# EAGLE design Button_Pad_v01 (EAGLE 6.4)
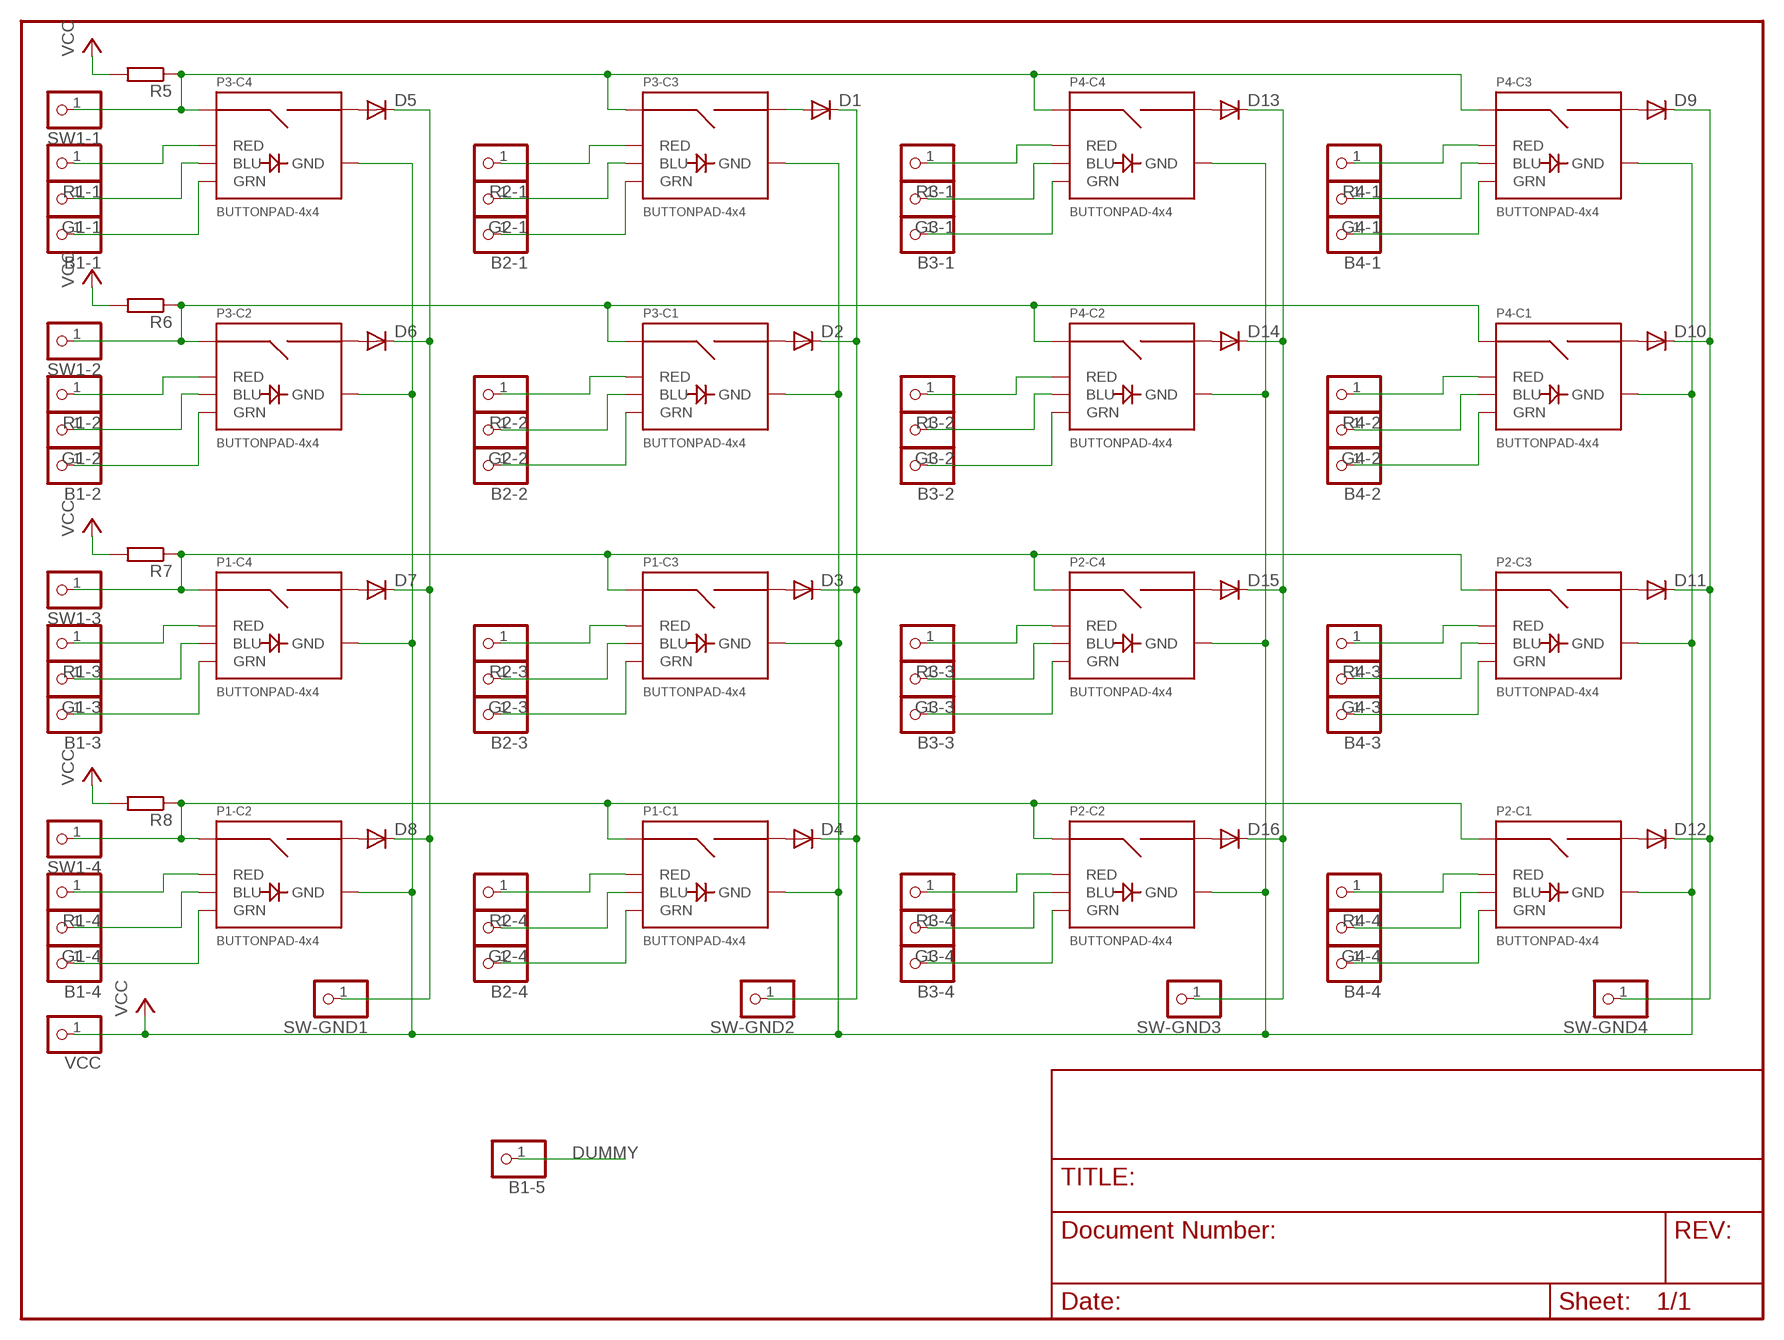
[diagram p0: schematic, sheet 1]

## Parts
B1-1  PINHD-1X1  [1X01]
B1-2  PINHD-1X1  [1X01]
B1-3  PINHD-1X1  [1X01]
B1-4  PINHD-1X1  [1X01]
B1-5  PINHD-1X1  [1X01]
B2-1  PINHD-1X1  [1X01]
B2-2  PINHD-1X1  [1X01]
B2-3  PINHD-1X1  [1X01]
B2-4  PINHD-1X1  [1X01]
B3-1  PINHD-1X1  [1X01]
B3-2  PINHD-1X1  [1X01]
B3-3  PINHD-1X1  [1X01]
B3-4  PINHD-1X1  [1X01]
B4-1  PINHD-1X1  [1X01]
B4-2  PINHD-1X1  [1X01]
B4-3  PINHD-1X1  [1X01]
B4-4  PINHD-1X1  [1X01]
D1  DIODE-1N4148  [DOIDE-1N4148]
D2  DIODE-1N4148  [DOIDE-1N4148]
D3  DIODE-1N4148  [DOIDE-1N4148]
D4  DIODE-1N4148  [DOIDE-1N4148]
D5  DIODE-1N4148  [DOIDE-1N4148]
D6  DIODE-1N4148  [DOIDE-1N4148]
D7  DIODE-1N4148  [DOIDE-1N4148]
D8  DIODE-1N4148  [DOIDE-1N4148]
D9  DIODE-1N4148  [DOIDE-1N4148]
D10  DIODE-1N4148  [DOIDE-1N4148]
D11  DIODE-1N4148  [DOIDE-1N4148]
D12  DIODE-1N4148  [DOIDE-1N4148]
D13  DIODE-1N4148  [DOIDE-1N4148]
D14  DIODE-1N4148  [DOIDE-1N4148]
D15  DIODE-1N4148  [DOIDE-1N4148]
D16  DIODE-1N4148  [DOIDE-1N4148]
G1-1  PINHD-1X1  [1X01]
G1-2  PINHD-1X1  [1X01]
G1-3  PINHD-1X1  [1X01]
G1-4  PINHD-1X1  [1X01]
G2-1  PINHD-1X1  [1X01]
G2-2  PINHD-1X1  [1X01]
G2-3  PINHD-1X1  [1X01]
G2-4  PINHD-1X1  [1X01]
G3-1  PINHD-1X1  [1X01]
G3-2  PINHD-1X1  [1X01]
G3-3  PINHD-1X1  [1X01]
G3-4  PINHD-1X1  [1X01]
G4-1  PINHD-1X1  [1X01]
G4-2  PINHD-1X1  [1X01]
G4-3  PINHD-1X1  [1X01]
G4-4  PINHD-1X1  [1X01]
P1  BUTTONPAD-4x4  BUTTONPAD-2X2  [BUTTONPAD-2X2]
P2  BUTTONPAD-4x4  BUTTONPAD-2X2  [BUTTONPAD-2X2]
P3  BUTTONPAD-4x4  BUTTONPAD-2X2  [BUTTONPAD-2X2]
P4  BUTTONPAD-4x4  BUTTONPAD-2X2  [BUTTONPAD-2X2]
R1-1  PINHD-1X1  [1X01]
R1-2  PINHD-1X1  [1X01]
R1-3  PINHD-1X1  [1X01]
R1-4  PINHD-1X1  [1X01]
R2-1  PINHD-1X1  [1X01]
R2-2  PINHD-1X1  [1X01]
R2-3  PINHD-1X1  [1X01]
R2-4  PINHD-1X1  [1X01]
R3-1  PINHD-1X1  [1X01]
R3-2  PINHD-1X1  [1X01]
R3-3  PINHD-1X1  [1X01]
R3-4  PINHD-1X1  [1X01]
R4-1  PINHD-1X1  [1X01]
R4-2  PINHD-1X1  [1X01]
R4-3  PINHD-1X1  [1X01]
R4-4  PINHD-1X1  [1X01]
R5  R-EU_0204/7  [0204/7]
R6  R-EU_0204/7  [0204/7]
R7  R-EU_0204/7  [0204/7]
R8  R-EU_0204/7  [0204/7]
SW1-1  PINHD-1X1  [1X01]
SW1-2  PINHD-1X1  [1X01]
SW1-3  PINHD-1X1  [1X01]
SW1-4  PINHD-1X1  [1X01]
SW-GND1  PINHD-1X1  [1X01]
SW-GND2  PINHD-1X1  [1X01]
SW-GND3  PINHD-1X1  [1X01]
SW-GND4  PINHD-1X1  [1X01]
VCC  PINHD-1X1  [1X01]

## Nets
DUMMY: B1-5.1
G3-2: G3-2.1 P4.BLU2(-C2:BLU)
N$1: D1.P$1(A) P3.SIG6(-C3:SIG2)
N$2: D2.P$1(A) P3.SIG2(-C1:SIG2)
N$3: D3.P$1(A) P1.SIG6(-C3:SIG2)
N$4: D4.P$1(A) P1.SIG2(-C1:SIG2)
N$5: D5.P$1(A) P3.SIG8(-C4:SIG2)
N$6: D6.P$1(A) P3.SIG4(-C2:SIG2)
N$7: D7.P$1(A) P1.SIG8(-C4:SIG2)
N$8: D8.P$1(A) P1.SIG4(-C2:SIG2)
N$9: D9.P$1(A) P4.SIG6(-C3:SIG2)
N$10: D10.P$1(A) P4.SIG2(-C1:SIG2)
N$11: D11.P$1(A) P2.SIG6(-C3:SIG2)
N$12: D12.P$1(A) P2.SIG2(-C1:SIG2)
N$13: D13.P$1(A) P4.SIG8(-C4:SIG2)
N$14: D14.P$1(A) P4.SIG4(-C2:SIG2)
N$15: D15.P$1(A) P2.SIG8(-C4:SIG2)
N$16: D16.P$1(A) P2.SIG4(-C2:SIG2)
N$17: B4-1.1 P4.GRN3(-C3:GRN)
N$18: G4-1.1 P4.BLU3(-C3:BLU)
N$19: P4.RED3(-C3:RED) R4-1.1
N$20: B4-2.1 P4.GRN1(-C1:GRN)
N$21: G4-2.1 P4.BLU1(-C1:BLU)
N$22: P4.RED1(-C1:RED) R4-2.1
N$23: P2.RED3(-C3:RED) R4-3.1
N$24: G4-3.1 P2.BLU3(-C3:BLU)
N$25: B4-3.1 P2.GRN3(-C3:GRN)
N$26: P3.RED4(-C4:RED) R1-1.1
N$27: B4-4.1 P2.GRN1(-C1:GRN)
N$28: G4-4.1 P2.BLU1(-C1:BLU)
N$29: P2.RED1(-C1:RED) R4-4.1
N$30: G1-1.1 P3.BLU4(-C4:BLU)
N$31: B1-1.1 P3.GRN4(-C4:GRN)
N$32: P2.RED2(-C2:RED) R3-4.1
N$33: B3-4.1 P2.GRN2(-C2:GRN)
N$34: G3-4.1 P2.BLU2(-C2:BLU)
N$35: B2-4.1 P1.GRN1(-C1:GRN)
N$36: G2-4.1 P1.BLU1(-C1:BLU)
N$37: P1.RED1(-C1:RED) R2-4.1
N$38: P1.RED2(-C2:RED) R1-4.1
N$39: G1-4.1 P1.BLU2(-C2:BLU)
N$40: B1-4.1 P1.GRN2(-C2:GRN)
N$41: B1-3.1 P1.GRN4(-C4:GRN)
N$42: G1-3.1 P1.BLU4(-C4:BLU)
N$43: P1.RED4(-C4:RED) R1-3.1
N$44: B1-2.1 P3.GRN2(-C2:GRN)
N$45: G1-2.1 P3.BLU2(-C2:BLU)
N$46: P3.RED2(-C2:RED) R1-2.1
N$47: P3.RED3(-C3:RED) R2-1.1
N$48: G2-1.1 P3.BLU3(-C3:BLU)
N$49: B2-1.1 P3.GRN3(-C3:GRN)
N$50: B2-2.1 P3.GRN1(-C1:GRN)
N$51: G2-2.1 P3.BLU1(-C1:BLU)
N$52: P3.RED1(-C1:RED) R2-2.1
N$53: B2-3.1 P1.GRN3(-C3:GRN)
N$54: G2-3.1 P1.BLU3(-C3:BLU)
N$55: P1.RED3(-C3:RED) R2-3.1
N$56: B3-3.1 P2.GRN4(-C4:GRN)
N$57: G3-3.1 P2.BLU4(-C4:BLU)
N$58: P2.RED4(-C4:RED) R3-3.1
N$59: B3-2.1 P4.GRN2(-C2:GRN)
N$61: P4.RED2(-C2:RED) R3-2.1
N$62: B3-1.1 P4.GRN4(-C4:GRN)
N$63: G3-1.1 P4.BLU4(-C4:BLU)
N$64: P4.RED4(-C4:RED) R3-1.1
SW2-1: P3.SIG5(-C3:SIG1) P3.SIG7(-C4:SIG1) P4.SIG5(-C3:SIG1) P4.SIG7(-C4:SIG1) R5.1 SW1-1.1
SW2-2: P3.SIG1(-C1:SIG1) P3.SIG3(-C2:SIG1) P4.SIG1(-C1:SIG1) P4.SIG3(-C2:SIG1) R6.1 SW1-2.1
SW2-3: P1.SIG5(-C3:SIG1) P1.SIG7(-C4:SIG1) P2.SIG5(-C3:SIG1) P2.SIG7(-C4:SIG1) R7.1 SW1-3.1
SW2-4: P1.SIG1(-C1:SIG1) P1.SIG3(-C2:SIG1) P2.SIG1(-C1:SIG1) P2.SIG3(-C2:SIG1) R8.1 SW1-4.1
SWT-GND1 [ButtonSignal]: D1.P$2(C) D2.P$2(C) D3.P$2(C) D4.P$2(C) SW-GND2.1
SWT-GND2 [ButtonSignal]: D5.P$2(C) D6.P$2(C) D7.P$2(C) D8.P$2(C) SW-GND1.1
SWT-GND3 [ButtonSignal]: D9.P$2(C) D10.P$2(C) D11.P$2(C) D12.P$2(C) SW-GND4.1
SWT-GND4 [ButtonSignal]: D13.P$2(C) D14.P$2(C) D15.P$2(C) D16.P$2(C) SW-GND3.1
VCC: P1.GND1(-C1:GND) P1.GND2(-C2:GND) P1.GND3(-C3:GND) P1.GND4(-C4:GND) P2.GND1(-C1:GND) P2.GND2(-C2:GND) P2.GND3(-C3:GND) P2.GND4(-C4:GND) P3.GND1(-C1:GND) P3.GND2(-C2:GND) P3.GND3(-C3:GND) P3.GND4(-C4:GND) P4.GND1(-C1:GND) P4.GND2(-C2:GND) P4.GND3(-C3:GND) P4.GND4(-C4:GND) R5.2 R6.2 R7.2 R8.2 VCC.1

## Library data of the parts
B1-1-B1-5 B2-1-B2-4 B3-1-B3-4 B4-1-B4-4 G1-1-G1-4 G2-1-G2-4 G3-1-G3-4 G4-1-G4-4 R1-1-R1-4 R2-1-R2-4 R3-1-R3-4 R4-1-R4-4 SW1-1-SW1-4 SW-GND1-SW-GND4 VCC = pinhead:PINHD-1X1: PIN HEADER
D1-D16 = SparkFun:DIODE-1N4148
P1-P4 = SparkFun:BUTTONPAD-2X2: 5mm Button Pad Proven layout and schematic for 2x2 button pad. Panelize this device/fp to a 4x4 pad if needed. Spark Fun Electronics SKU : COM-07835. Compatible common cathode tri-color LED SKU : COM-00105
R5-R8 = rcl:R-EU_: RESISTOR, European symbol

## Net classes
0 Default: width 0.254 mm, clearance 0.355 mm
1 Power: width 0.305 mm
2 LEDPower: width 0.305 mm
3 ButtonSignal: width 0.254 mm, clearance 0.355 mm to class 0, clearance 0.355 mm to class 1, clearance 0.355 mm to class 2, clearance 0.355 mm

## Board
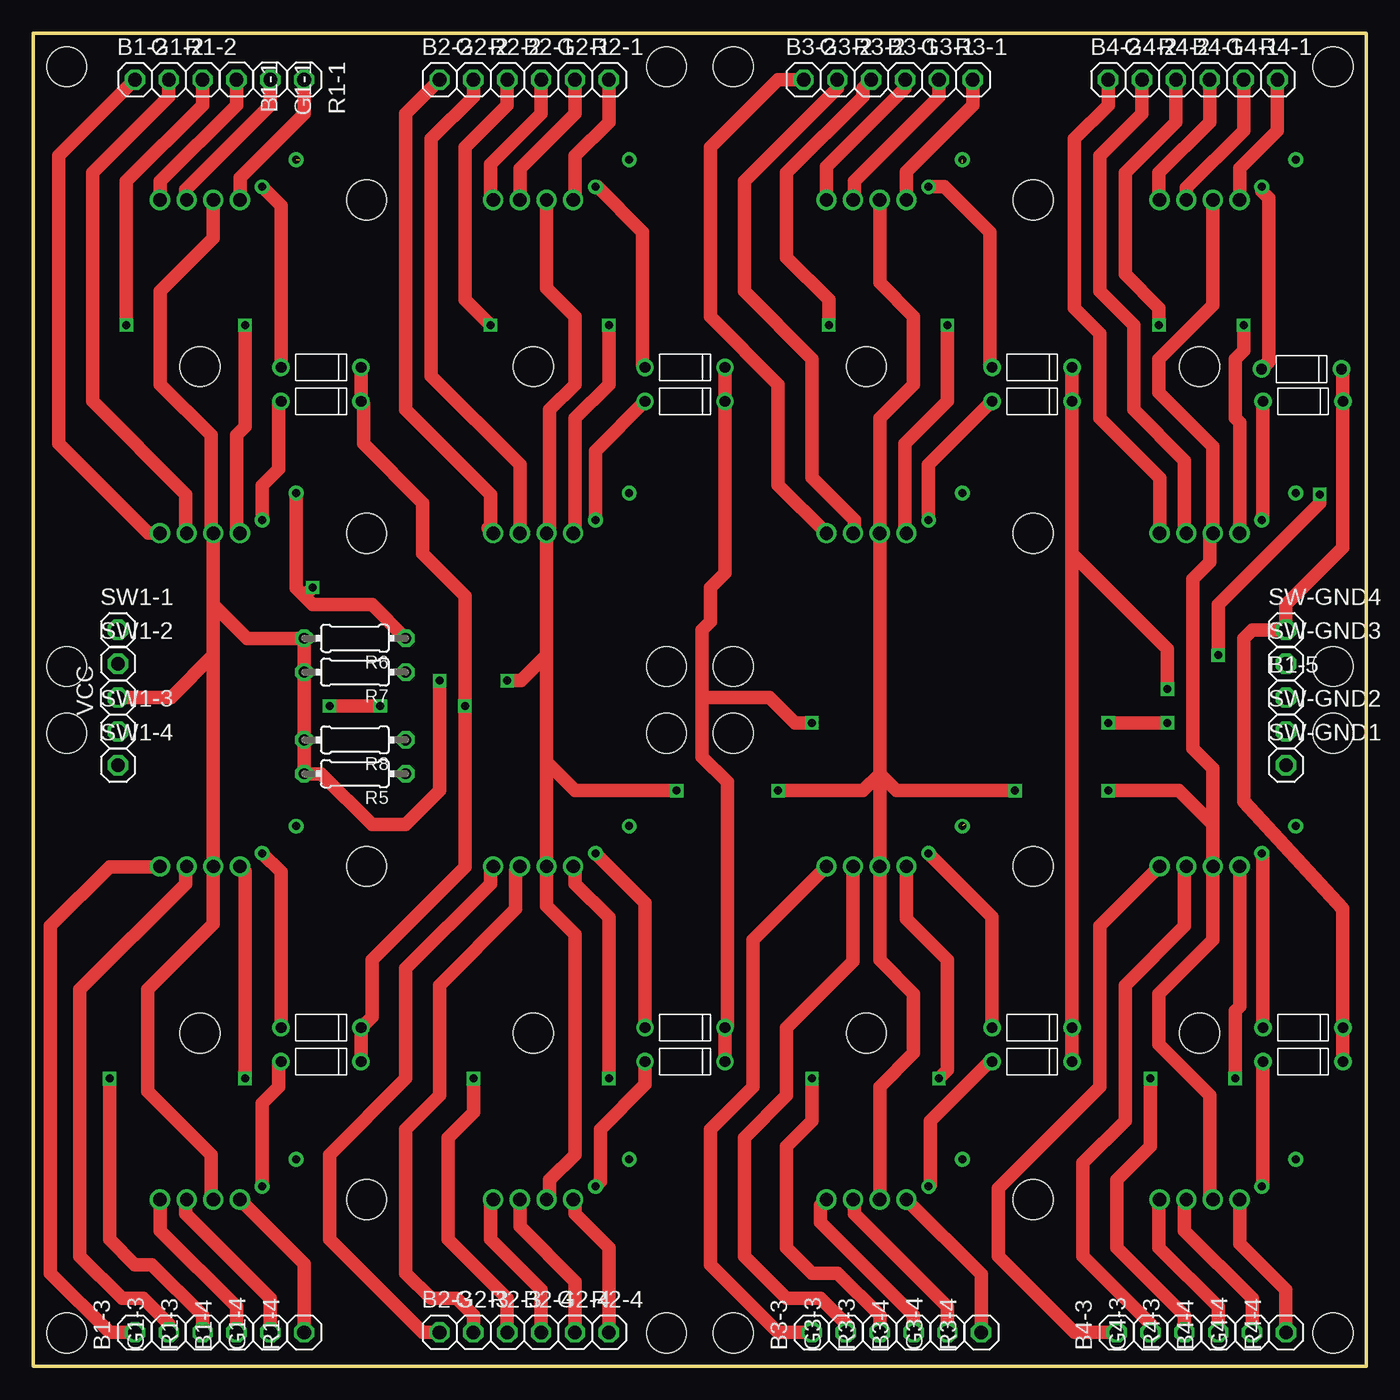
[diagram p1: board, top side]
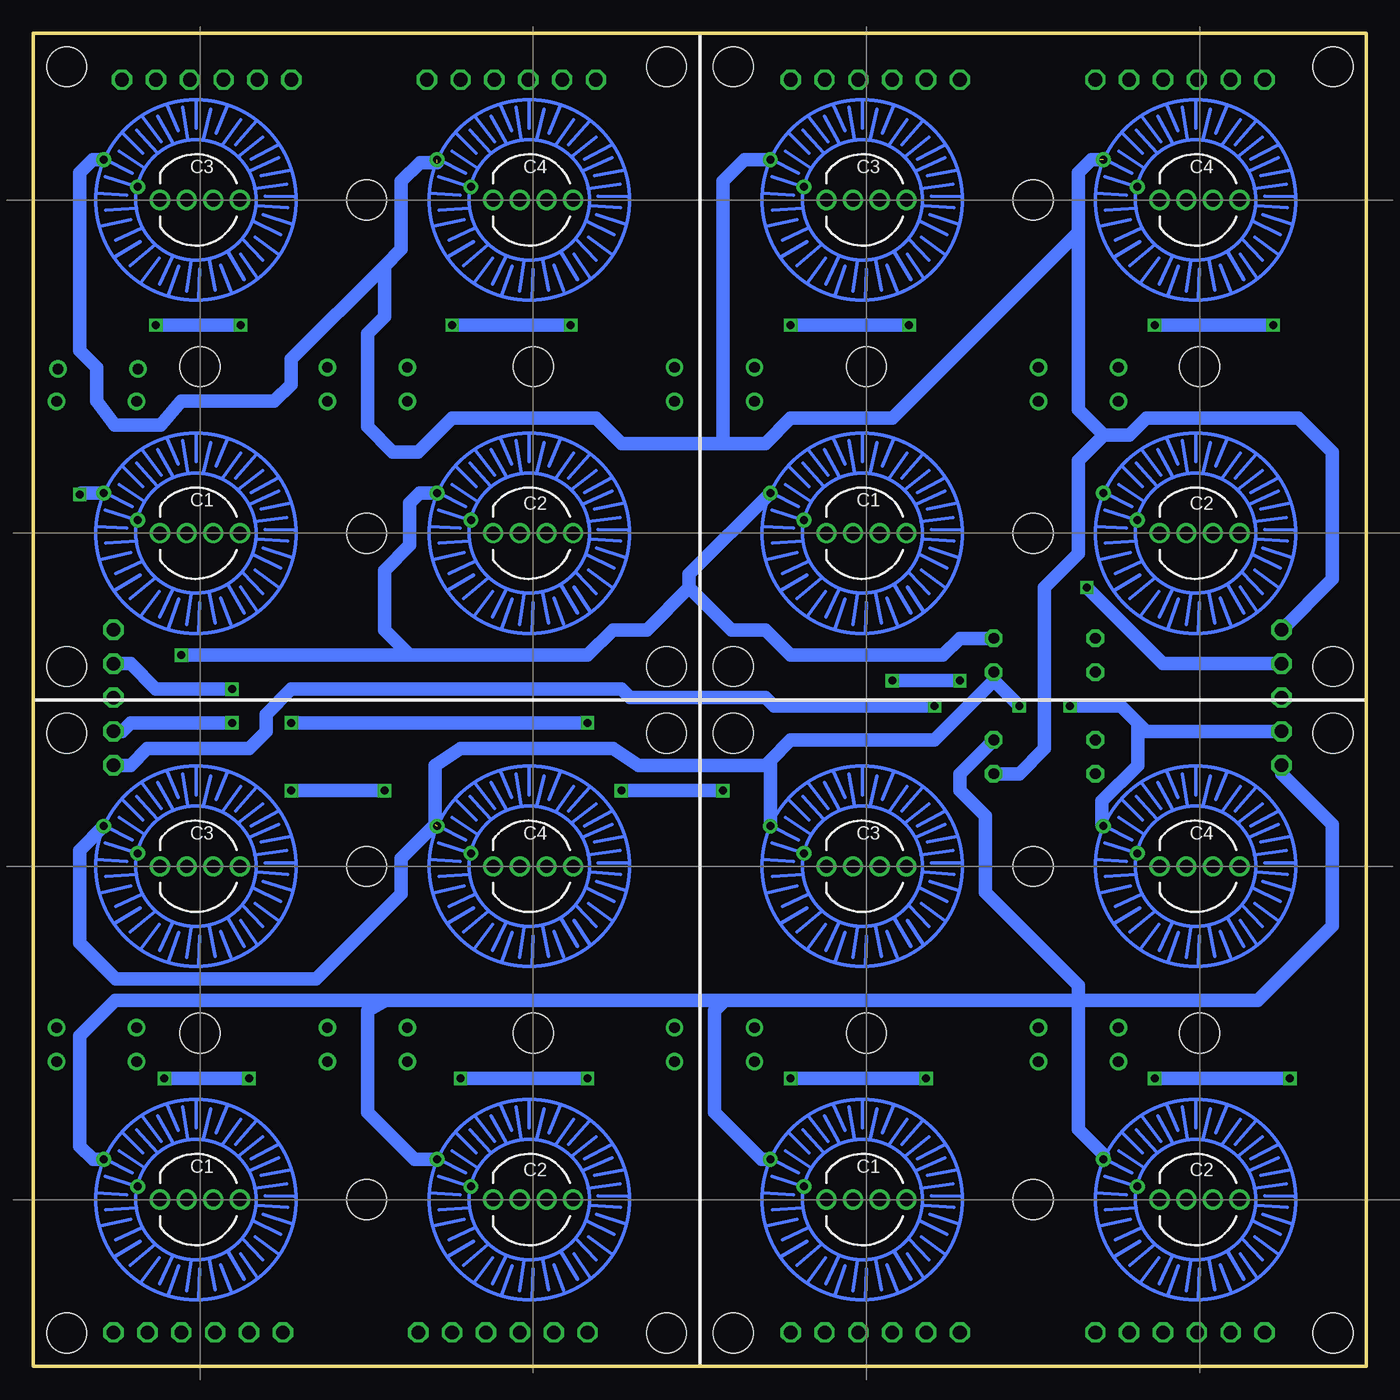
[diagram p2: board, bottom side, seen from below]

Size 100 x 100 mm. Coordinates in mm from the lower left corner, seen from the top.
Outline: 0,0 100,0 100,100 0,100 0,0
Copper layers (1*16): Top 0.035mm / dielectric 1.5mm / Bottom 0.035mm
Design rules "default *": minimum track width 7mil, minimum drill 20mil, track to track 7mil, track to pad 7mil, pad to pad 7mil, via to via 7mil, smd to smd 7mil, copper to edge 20mil, drill to drill 7mil, minimum pad ring 10mil, minimum via ring 8mil, stop-mask expansion 4mil, vias tented up to drill 0mil, thermal gap 10mil

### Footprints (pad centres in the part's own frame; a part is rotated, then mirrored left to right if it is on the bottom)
1X01 = drill 1.016 octagon: 1 0,0
DOIDE-1N4148 = drill 0.8: P$1 3,0; P$2 -3,0
BUTTONPAD-2X2 = drill 1: BLU1 13.5,12.5; BLU2 38.5,12.5; BLU3 13.5,37.5; BLU4 38.5,37.5; GND1 11.5,12.5; GND2 36.5,12.5; GND3 11.5,37.5; GND4 36.5,37.5; GRN1 15.5,12.5; GRN2 40.5,12.5; GRN3 15.5,37.5; GRN4 40.5,37.5; RED1 9.5,12.5; RED2 34.5,12.5; RED3 9.5,37.5; RED4 34.5,37.5 | drill 0.6: SIG1 5.288,15.513; SIG2 7.828,13.481; SIG3 30.288,15.513; SIG4 32.828,13.481; SIG5 5.288,40.513; SIG6 7.828,38.481; SIG7 30.288,40.513; SIG8 32.828,38.481 | hole 3: 12.5,25; 25,37.5; 37.5,25; 25,12.5; 2.5,2.5; 2.5,47.5; 47.5,47.5; 47.5,2.5
0204/7 = drill 0.813 octagon: 1 -3.81,0; 2 3.81,0

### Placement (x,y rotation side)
B1-1  15.24,96.52 270 top
B1-2  7.62,96.52 0 top
B1-3  7.62,2.54 90 top
B1-4  15.24,2.54 90 top
B1-5  93.98,50.16 0 top
B2-1  38.1,96.52 0 top
B2-2  30.48,96.52 0 top
B2-3  30.48,2.54 0 top
B2-4  38.1,2.54 0 top
B3-1  65.41,96.52 0 top
B3-2  57.78,96.52 0 top
B3-3  58.42,2.54 90 top
B3-4  66.04,2.54 90 top
B4-1  88.27,96.52 0 top
B4-2  80.64,96.52 0 top
B4-3  81.28,2.54 90 top
B4-4  88.9,2.54 90 top
D1  48.9,74.93 180 top
D2  48.9,72.39 180 top
D3  48.9,25.4 180 top
D4  48.9,22.86 180 top
D5  21.59,74.93 180 top
D6  21.59,72.39 180 top
D7  21.59,25.4 180 top
D8  21.59,22.86 180 top
D9  95.15,74.81 180 top
D10  95.25,72.39 180 top
D11  95.25,25.4 180 top
D12  95.25,22.86 180 top
D13  74.93,74.93 180 top
D14  74.93,72.39 180 top
D15  74.93,25.4 180 top
D16  74.93,22.86 180 top
G1-1  17.78,96.52 270 top
G1-2  10.16,96.52 0 top
G1-3  10.16,2.54 90 top
G1-4  17.78,2.54 90 top
G2-1  40.64,96.52 0 top
G2-2  33.02,96.52 0 top
G2-3  33.02,2.54 0 top
G2-4  40.64,2.54 0 top
G3-1  67.94,96.52 0 top
G3-2  60.33,96.52 0 top
G3-3  60.96,2.54 90 top
G3-4  68.58,2.54 90 top
G4-1  90.81,96.52 0 top
G4-2  83.19,96.52 0 top
G4-3  83.82,2.54 90 top
G4-4  91.44,2.54 90 top
P1  50,0 0 bottom
P2  100,0 0 bottom
P3  50,50 0 bottom
P4  100,50 0 bottom
R1-1  20.32,96.52 270 top
R1-2  12.7,96.52 0 top
R1-3  12.7,2.54 90 top
R1-4  20.32,2.54 90 top
R2-1  43.18,96.52 0 top
R2-2  35.56,96.52 0 top
R2-3  35.56,2.54 0 top
R2-4  43.18,2.54 0 top
R3-1  70.48,96.52 0 top
R3-2  62.87,96.52 0 top
R3-3  63.5,2.54 90 top
R3-4  71.12,2.54 90 top
R4-1  93.34,96.52 0 top
R4-2  85.72,96.52 0 top
R4-3  86.36,2.54 90 top
R4-4  93.98,2.54 90 top
R5  24.13,44.45 180 top
R6  24.13,54.61 180 top
R7  24.13,52.07 180 top
R8  24.13,46.99 180 top
SW1-1  6.35,55.24 0 top
SW1-2  6.35,52.7 0 top
SW1-3  6.35,47.62 0 top
SW1-4  6.35,45.09 0 top
SW-GND1  93.98,45.09 0 top
SW-GND2  93.98,47.62 0 top
SW-GND3  93.98,52.7 0 top
SW-GND4  93.98,55.24 0 top
VCC  6.35,50.16 90 top

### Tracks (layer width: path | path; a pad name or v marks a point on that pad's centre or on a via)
G3-2
  Top 1.016: P4.BLU2 61.59,62.59 61.59,63.5 58.42,66.67 58.42,75.56 53.34,80.64 53.34,88.9 60.33,95.89 G3-2.1
N$1
  Top 1.016: P3.SIG6 42.33,88.48 45.72,85.09 45.72,75.11 D1.P$1
N$2
  Top 1.016: P3.SIG2 42.17,68.67 D2.P$1
N$3
  Top 1.016: D3.P$1 45.9,34.76 P1.SIG6
N$4
  Top 1.016: D4.P$1 45.9,21.13 42.55,17.78 42.55,13.85 P1.SIG2
N$5
  Top 1.016: D5.P$1 18.59,87.06 P3.SIG8
N$6
  Top 1.016: P3.SIG4 17.17,66.07 18.41,67.31 18.41,72.22 D6.P$1
N$7
  Top 1.016: D7.P$1 18.59,37.06 P1.SIG8
N$8
  Top 1.016: P1.SIG4 17.17,19.71 18.41,20.95 18.41,22.68 D8.P$1
N$9
  Top 1.016: P4.SIG6 92.17,88.17 92.71,87.63 92.71,75.37 D9.P$1
N$10
  Top 1.016: D10.P$1 92.25,63.56 P4.SIG2
N$11
  Top 1.016: D11.P$1 92.25,38.4 P2.SIG6
N$12
  Top 1.016: D12.P$1 92.25,13.56 P2.SIG2
N$13
  Top 1.016: P4.SIG8 68.36,88.48 71.75,85.09 71.75,75.11 D13.P$1
N$14
  Top 1.016: P4.SIG4 67.17,67.63 D14.P$1
N$15
  Top 1.016: D15.P$1 71.93,33.72 P2.SIG8
N$16
  Top 1.016: D16.P$1 71.75,22.86 67.31,18.41 67.31,13.62 P2.SIG4
N$17
  Top 1.016: B4-1.1 88.27,93.34 84.45,89.53 84.45,87.55 P4.GRN3
N$18
  Top 1.016: P4.BLU3 86.5,88.41 90.81,92.71 G4-1.1
N$19
  Top 1.016: P4.RED3 90.5,89.86 93.34,92.71 R4-1.1
N$20
  Top 1.016: P4.GRN1 84.5,66.63 80.01,71.12 80.01,77.47 78.11,79.38 78.11,92.08 80.64,94.61 B4-2.1
N$21
  Top 1.016: P4.BLU1 86.36,62.64 86.36,67.94 82.55,71.75 82.55,78.11 80.01,80.64 80.01,90.81 83.19,93.98 G4-2.1
N$22  (via drill 0.6)
  Top 1.016: R4-2.1 85.72,93.34 81.92,89.53 81.92,81.92 84.45,79.38 v84.45,78.11 | v90.81,78.11 90.81,76.2 90.17,75.56 90.17,71.12 90.5,70.79 P4.RED1
  Bottom 1.016: v84.45,78.11 v90.81,78.11
N$23  (via drill 0.6)
  Top 1.016: R4-3.1 86.36,3.81 81.28,8.89 81.28,13.97 83.82,16.51 v83.82,21.59 | P2.RED3 90.5,27 90.17,26.67 v90.17,21.59
  Bottom 1.016: v83.82,21.59 v90.17,21.59
N$24
  Top 1.016: G4-3.1 83.82,3.17 78.74,8.26 78.74,15.24 81.92,18.41 81.92,28.57 86.36,33.02 86.36,37.36 P2.BLU3
N$25
  Top 1.016: P2.GRN3 80.01,33.02 80.01,20.95 72.39,13.34 72.39,8.26 78.11,2.54 B4-3.1
N$26
  Top 1.016: R1-1.1 20.32,93.98 15.5,89.16 P3.RED4
N$27
  Top 1.016: P2.GRN1 84.45,12.46 84.45,8.89 88.9,4.45 B4-4.1
N$28
  Top 1.016: G4-4.1 91.44,5.08 86.36,10.16 86.36,12.36 P2.BLU1
N$29
  Top 1.016: R4-4.1 93.98,5.71 90.5,9.2 P2.RED1
N$30
  Top 1.016: G1-1.1 17.78,94.61 11.43,88.27 11.43,87.57 P3.BLU4
N$31
  Top 1.016: P3.GRN4 9.53,87.53 9.53,88.9 15.24,94.61 B1-1.1
N$32
  Top 1.016: R3-4.1 71.12,6.88 P2.RED2
N$33
  Top 1.016: B3-4.1 66.04,3.81 59.05,10.79 59.05,12.05 P2.GRN2
N$34
  Top 1.016: G3-4.1 68.58,4.45 61.59,11.43 61.59,12.4 P2.BLU2
N$35
  Top 1.016: B2-4.1 38.1,5.71 34.29,9.53 34.29,12.29 P1.GRN1
N$36
  Top 1.016: G2-4.1 40.64,6.35 36.5,10.49 P1.BLU1
N$37
  Top 1.016: R2-4.1 43.18,8.89 40.64,11.43 40.64,12.36 P1.RED1
N$38
  Top 1.016: R1-4.1 20.32,7.68 P1.RED2
N$39
  Top 1.016: G1-4.1 17.78,5.08 11.43,11.43 11.43,12.43 P1.BLU2
N$40
  Top 1.016: B1-4.1 15.24,4.45 9.53,10.16 9.53,12.47 P1.GRN2
N$41
  Top 1.016: B1-3.1 5.71,2.54 1.27,6.99 1.27,33.02 5.71,37.47 9.46,37.47 P1.GRN4
N$42
  Top 1.016: P1.BLU4 11.43,37.43 11.43,36.2 3.49,28.26 3.49,8.26 6.67,5.08 8.26,5.08 10.16,3.17 G1-3.1
N$43  (via drill 0.6)
  Top 1.016: R1-3.1 12.7,3.81 8.89,7.62 7.62,7.62 5.71,9.53 v5.71,21.59 | v15.88,21.59 15.88,37.12 P1.RED4
  Bottom 1.016: v5.71,21.59 v15.88,21.59
N$44
  Top 1.016: P3.GRN2 8.62,62.5 1.91,69.22 1.91,90.81 B1-2.1
N$45
  Top 1.016: G1-2.1 10.16,95.25 4.45,89.53 4.45,72.39 11.43,65.41 11.43,62.57 P3.BLU2
N$46  (via drill 0.6)
  Top 1.016: P3.RED2 15.24,62.76 15.24,69.85 15.88,70.48 v15.88,78.11 | R1-2.1 12.7,94.61 6.99,88.9 v6.99,78.11
  Bottom 1.016: v6.99,78.11 v15.88,78.11
N$47
  Top 1.016: R2-1.1 43.18,93.34 40.64,90.81 40.64,87.64 P3.RED3
N$48
  Top 1.016: P3.BLU3 36.5,89.84 40.64,93.98 G2-1.1
N$49
  Top 1.016: B2-1.1 38.1,93.98 34.29,90.17 34.29,87.71 P3.GRN3
N$50
  Top 1.016: B2-2.1 27.94,93.98 27.94,71.75 34.29,65.41 34.29,63.02 34.13,62.87 P3.GRN1
N$51
  Top 1.016: P3.BLU1 36.5,67.64 29.84,74.3 29.84,92.08 33.02,95.25 G2-2.1
N$52  (via drill 0.6)
  Top 1.016: R2-2.1 35.56,94.61 32.38,91.44 32.38,80.01 v34.29,78.11 | v43.18,78.11 43.18,73.66 40.64,71.12 40.64,62.64 P3.RED1
  Bottom 1.016: v34.29,78.11 v43.18,78.11
N$53
  Top 1.016: P1.GRN3 34.29,37.29 34.29,36.2 27.94,29.84 27.94,21.59 22.23,15.88 22.23,9.53 29.21,2.54 B2-3.1
N$54
  Top 1.016: G2-3.1 33.02,3.81 31.75,5.08 29.84,5.08 27.94,6.99 27.94,17.78 30.48,20.32 30.48,28.57 36.2,34.29 36.2,37.2 P1.BLU3
N$55  (via drill 0.6)
  Top 1.016: v33.02,21.59 33.02,19.05 31.11,17.14 31.11,9.53 35.56,5.08 R2-3.1 | P1.RED3 40.64,37.36 40.64,36.2 43.18,33.66 v43.18,21.59
  Bottom 1.016: v33.02,21.59 v43.18,21.59
N$56
  Top 1.016: B3-3.1 55.88,2.54 50.8,7.62 50.8,17.78 53.98,20.95 53.98,31.98 P2.GRN4
N$57
  Top 1.016: G3-3.1 60.96,3.17 59.05,5.08 56.52,5.08 53.34,8.26 53.34,17.14 56.52,20.32 56.52,25.4 61.5,30.39 P2.BLU4
N$58  (via drill 0.6)
  Top 1.016: R3-3.1 63.5,3.81 60.33,6.99 58.42,6.99 56.52,8.89 56.52,16.51 58.42,18.41 v58.42,21.59 | P2.RED4 65.5,33.56 68.58,30.48 68.58,22.23 v67.94,21.59
  Bottom 1.016: v58.42,21.59 v67.94,21.59
N$59
  Top 1.016: B3-2.1 55.88,96.52 50.8,91.44 50.8,78.74 55.88,73.66 55.88,66.12 P4.GRN2
N$61  (via drill 0.6)
  Top 1.016: P4.RED2 65.41,62.59 65.41,69.22 68.58,72.39 v68.58,78.11 | R3-2.1 62.23,95.89 62.23,95.25 56.52,89.53 56.52,83.19 59.69,80.01 v59.69,78.11
  Bottom 1.016: v59.69,78.11 v68.58,78.11
N$62
  Top 1.016: P4.GRN4 59.5,89.98 65.41,95.89 B3-1.1
N$63
  Top 1.016: G3-1.1 67.94,95.25 61.59,88.9 61.59,87.59 P4.BLU4
N$64
  Top 1.016: P4.RED4 65.5,89.63 70.48,94.61 R3-1.1
SW2-1  (2 unrouted)
  Bottom 1.016: P3.SIG5 46.65,90.51 48.26,88.9 48.26,69.22 | 73.66,82.55 80.64,75.56 80.64,73.66 81.92,72.39 88.9,72.39 90.43,70.62 93.9,70.62 95.25,72.39 95.25,74.93 96.52,76.2 96.52,89.53 95.54,90.51 P4.SIG5 | 73.66,82.55 73.66,78.74 74.93,77.47 74.93,70.48 73.03,68.58 71.12,68.58 68.58,71.12 57.78,71.12 55.88,69.22 48.26,69.22 | 19.68,69.85 17.78,69.85 16.51,71.12 5.08,71.12 2.54,68.58 2.54,59.05 SW1-1.1 | 19.68,69.85 21.59,71.75 21.59,85.09 | 48.26,69.22 45.09,69.22 43.18,71.12 35.56,71.12 21.59,85.09 | 19.68,69.85 21.59,67.94 21.59,60.96 24.13,58.42 24.13,46.35 26.04,44.45 R5.1 | 21.59,85.09 21.59,89.53 20.61,90.51 19.98,90.51 | 69.71,90.31 70.98,90.31 72.39,88.9 72.39,83.82 73.66,82.55
SW2-2  (via drill 0.6)
  Top 1.016: P3.SIG3 19.71,58.39 20.32,57.78 | 20.32,57.78 20.95,57.15 25.4,57.15 R6.1 | v20.95,58.42 20.32,57.78 | v88.9,53.34 88.9,57.15 96.52,64.77 v96.52,65.41
  Bottom 1.016: P3.SIG1 50.8,59.42 50.8,58.42 | 50.8,58.42 47.62,55.24 45.09,55.24 43.18,53.34 31.75,53.34 30.48,54.61 R6.1 | 50.8,58.42 53.98,55.24 56.52,55.24 58.42,53.34 71.75,53.34 | P4.SIG3 71.01,65.51 71.75,64.77 71.75,61.59 73.66,59.69 73.66,55.24 71.75,53.34 | v20.95,58.42 15.24,52.7 SW1-2.1 | 71.75,53.34 v88.9,53.34 | P4.SIG1 96.41,65.51 v96.52,65.41
SW2-3  (via drill 0.6)  (1 unrouted)
  Top 1.016: v22.23,49.53 v26.04,49.53
  Bottom 1.016: 19.68,40.54 P1.SIG7 19.84,40.64 19.84,42.39 17.14,45.09 17.14,48.26 | 69.85,40.65 69.85,45.09 67.94,46.35 56.52,46.35 54.61,45.09 45.09,45.09 44.71,45.46 | P1.SIG5 44.71,45.46 | 44.71,45.46 43.18,46.99 32.38,46.99 27.94,51.44 | 27.94,51.44 R7.1 | 17.14,48.26 18.41,49.53 v22.23,49.53 | v26.04,49.53 27.94,51.44 | P2.SIG7 69.98,40.51 72.39,38.1 72.39,35.42 78.76,29.04 93.81,29.04 96.52,31.75 96.52,38.7 P2.SIG5 | SW1-3.1 16.51,47.62 17.14,48.26
SW2-4
  Bottom 1.016: P1.SIG1 45.36,15.51 48.9,19.05 48.9,26.67 48.12,27.44 | P2.SIG3 71.39,15.51 74.93,19.05 74.93,26.67 73.54,27.44 | 73.54,27.44 93.86,27.44 96.52,24.78 96.52,16.51 95.52,15.51 P2.SIG1 | P1.SIG3 19.71,15.9 21.59,17.78 21.59,27.44 | R8.1 30.48,44.45 30.48,43.18 28.57,41.27 28.57,35.56 21.59,28.57 21.59,27.44 | 73.54,27.44 48.12,27.44 | 48.12,27.44 21.59,27.44 | 21.59,27.44 8.12,27.44 2.54,33.02 2.54,40.64 6.35,44.45 SW1-4.1
SWT-GND1  (via drill 0.6)
  Top 1.016: D1.P$2 D2.P$2 51.9,59.52 50.8,58.42 50.8,55.88 50.16,55.24 50.16,50.16 | D4.P$2 D3.P$2 52.07,25.57 52.07,43.81 50.16,45.72 50.16,50.16 | 50.16,50.16 55.24,50.16 57.15,48.26 v58.42,48.26 | v80.64,48.26 v85.09,48.26
  Bottom 1.016: v80.64,48.26 v58.42,48.26 | SW-GND2.1 93.34,47.62 92.71,48.26 v85.09,48.26
SWT-GND2  (via drill 0.6)
  Top 1.016: D5.P$2 D6.P$2 24.77,72.22 24.77,69.22 29.21,64.77 29.21,60.96 32.38,57.78 v32.38,49.53 32.38,37.47 25.4,30.48 25.4,26.21 D7.P$2 D8.P$2
  Bottom 1.016: v32.38,49.53 44.45,49.53 45.09,50.16 55.24,50.16 55.88,50.8 80.64,50.8 82.55,48.9 82.55,47.62 83.82,46.35 91.44,46.35 92.71,45.09 SW-GND1.1
SWT-GND3
  Top 1.016: D9.P$2 98.25,74.71 D10.P$2 98.25,61.42 93.98,57.15 SW-GND4.1 91.44,55.24 90.81,54.61 90.81,42.37 98.25,34.29 D11.P$2 D12.P$2
SWT-GND4  (via drill 0.6)
  Top 1.016: D13.P$2 D14.P$2 77.93,60.96 | D16.P$2 D15.P$2 77.93,60.96 | v85.09,50.8 85.09,53.8 77.93,60.96
  Bottom 1.016: v85.09,50.8 90.81,50.8 92.71,52.7 SW-GND3.1
VCC  (via drill 0.6)
  Top 1.016: 38.5,53.34 P3.GND1 38.73,62.73 38.73,71.75 40.64,73.66 40.64,78.74 38.5,80.88 P3.GND3 | 38.5,53.34 38.5,45.32 | 38.5,45.32 P1.GND3 38.5,34.52 40.64,32.38 40.64,15.88 38.73,13.97 38.73,12.73 P1.GND1 | 13.5,53.34 P1.GND4 13.5,33.19 8.57,28.26 8.57,20.64 13.34,15.88 13.34,12.66 P1.GND2 | 13.5,53.34 13.5,57.15 | 13.5,57.15 P3.GND2 13.34,62.66 13.34,69.85 9.53,73.66 9.53,80.64 13.5,84.62 P3.GND4 | 63.5,44.45 P4.GND2 63.5,71.12 66.04,73.66 66.04,78.74 63.5,81.28 P4.GND4 | 63.5,44.45 P2.GND4 63.5,30.48 66.04,27.94 66.04,23.5 63.5,20.95 P2.GND2 | 38.5,45.32 40.64,43.18 v48.26,43.18 | v55.88,43.18 62.23,43.18 63.5,44.45 | 63.5,44.45 64.77,43.18 v73.66,43.18 | P4.GND3 88.5,79.61 84.45,75.56 84.45,73.03 88.5,68.98 P4.GND1 88.27,62.27 88.27,60.33 87,59.05 87,46.35 88.5,44.85 88.5,40.64 | P2.GND1 88.27,12.73 88.27,20.32 84.45,24.13 84.45,27.94 88.5,31.98 P2.GND3 88.5,40.64 | 13.5,57.15 16.04,54.61 R6.2 R7.2 R8.2 R5.2 21.59,44.45 25.4,40.64 27.94,40.64 30.48,43.18 v30.48,51.44 | v35.56,51.44 36.59,51.44 38.5,53.34 | v80.64,43.18 85.96,43.18 88.5,40.64 | VCC.1 10.32,50.16 13.5,53.34
  Bottom 1.016: v48.26,43.18 v55.88,43.18 | v73.66,43.18 v80.64,43.18 | v30.48,51.44 v35.56,51.44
